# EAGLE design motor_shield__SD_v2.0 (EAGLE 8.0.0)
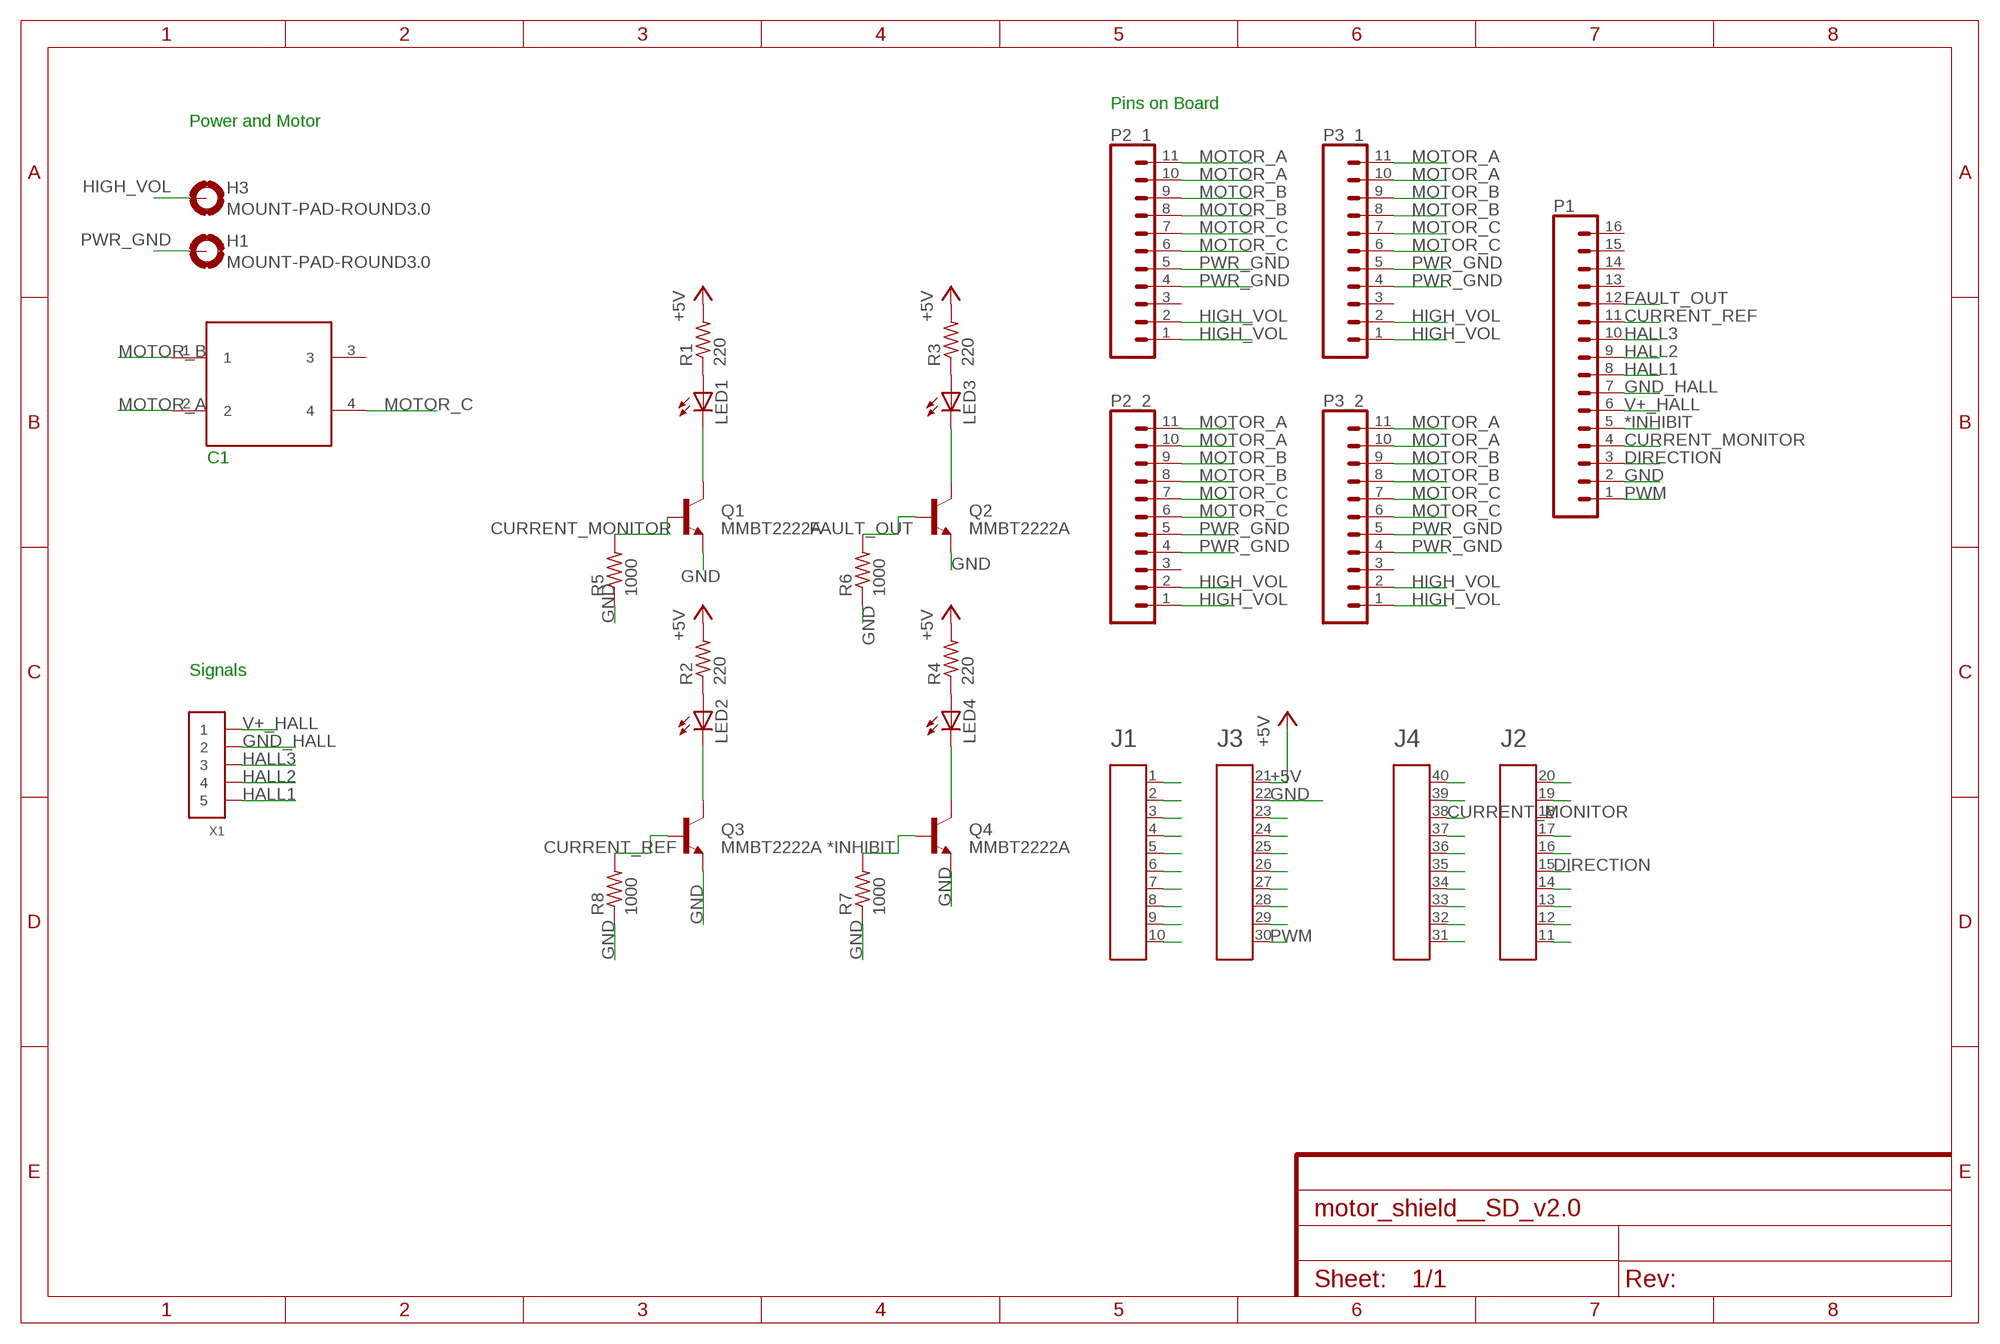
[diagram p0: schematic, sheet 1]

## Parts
A1  HEADER4X10-BOOSTERPACK  [4X10-BOOSTERPACK]
C1  MOLEX4CON  [MOLEX4CON]
H1  MOUNT-PAD-ROUND3.0  [3,0-PAD]
H3  MOUNT-PAD-ROUND3.0  [3,0-PAD]
LED1  LEDCHIPLED_0805  [CHIPLED_0805]
LED2  LEDCHIPLED_0805  [CHIPLED_0805]
LED3  LEDCHIPLED_0805  [CHIPLED_0805]
LED4  LEDCHIPLED_0805  [CHIPLED_0805]
P1  CONN_16LOCK  [1X16_LOCK]
P2_1  CONN_11  [1X11]
P2_2  CONN_11  [1X11]
P3_1  CONN_11  [1X11]
P3_2  CONN_11  [1X11]
Q1  MMBT2222A  TRANSISTOR_NPNMMBT2222A  [SOT23-3]
Q2  MMBT2222A  TRANSISTOR_NPNMMBT2222A  [SOT23-3]
Q3  MMBT2222A  TRANSISTOR_NPNMMBT2222A  [SOT23-3]
Q4  MMBT2222A  TRANSISTOR_NPNMMBT2222A  [SOT23-3]
R1  220  R-US_R0603  [R0603]
R2  220  R-US_R0603  [R0603]
R3  220  R-US_R0603  [R0603]
R4  220  R-US_R0603  [R0603]
R5  1000  R-US_R0603  [R0603]
R6  1000  R-US_R0603  [R0603]
R7  1000  R-US_R0603  [R0603]
R8  1000  R-US_R0603  [R0603]
X1  CONN_5-1-53261  [PB-53261-05]

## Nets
*INHIBIT: P1.5 Q4.1(B) R7.2
+5V: A1.21 R1.2 R2.2 R3.2 R4.2
CURRENT_MONITOR: A1.38 P1.4 Q1.1(B) R5.2
CURRENT_REF: P1.11 Q3.1(B) R8.2
DIRECTION: A1.15 P1.3
FAULT_OUT: P1.12 Q2.1(B) R6.2
GND: A1.22 P1.2 Q1.2(E) Q2.2(E) Q3.2(E) Q4.2(E) R5.1 R6.1 R7.1 R8.1
GND_HALL: P1.7 X1.2
HALL1: P1.8 X1.5
HALL2: P1.9 X1.4
HALL3: P1.10 X1.3
HIGH_VOL: H3.B3,0(MOUNT) P2_1.1 P2_1.2 P2_2.1 P2_2.2 P3_1.1 P3_1.2 P3_2.1 P3_2.2
MOTOR_A: C1.2 P2_1.10 P2_1.11 P2_2.10 P2_2.11 P3_1.10 P3_1.11 P3_2.10 P3_2.11
MOTOR_B: C1.1 P2_1.8 P2_1.9 P2_2.8 P2_2.9 P3_1.8 P3_1.9 P3_2.8 P3_2.9
MOTOR_C: C1.4 P2_1.6 P2_1.7 P2_2.6 P2_2.7 P3_1.6 P3_1.7 P3_2.6 P3_2.7
N$1: LED1.A R1.1
N$2: LED2.A R2.1
N$10: LED3.A R3.1
N$11: LED4.A R4.1
N$15: LED1.C Q1.3(C)
N$16: LED2.C Q3.3(C)
N$30: LED3.C Q2.3(C)
N$41: LED4.C Q4.3(C)
N$46: A1.1
N$47: A1.2
N$48: A1.3
N$49: A1.4
N$50: A1.5
N$51: A1.6
N$52: A1.7
N$53: A1.8
N$54: A1.9
N$55: A1.10
N$58: A1.23
N$59: A1.24
N$60: A1.25
N$61: A1.26
N$62: A1.27
N$63: A1.28
N$64: A1.29
N$66: A1.40
N$67: A1.39
N$69: A1.37
N$70: A1.36
N$71: A1.35
N$72: A1.34
N$73: A1.33
N$74: A1.32
N$75: A1.31
N$76: A1.20
N$77: A1.19
N$79: A1.17
N$80: A1.16
N$82: A1.14
N$83: A1.13
N$84: A1.12
N$85: A1.11
PWM: A1.30 P1.1
PWR_GND: H1.B3,0(MOUNT) P2_1.4 P2_1.5 P2_2.4 P2_2.5 P3_1.4 P3_1.5 P3_2.4 P3_2.5
V+_HALL: P1.6 X1.1
Unconnected: A1.18 C1.3 P1.13 P1.14 P1.15 P1.16 P2_1.3 P2_2.3 P3_1.3 P3_2.3

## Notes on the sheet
- Pins on Board
- Power and Motor
- C1
- Signals

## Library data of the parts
A1 = EAGLE_BoosterPack_Library:HEADER4X10-BOOSTERPACK
C1 = TREC1:MOLEX4CON
H1 H3 = holes:MOUNT-PAD-ROUND: MOUNTING PAD, round
LED1-LED4 = adafruit:LED: LED
P1 = SparkFun-Connectors:CONN_16: Multi connection point. Often used as Generic Header-pin footprint for 0.1 inch spaced/style header connections On any of the 0.1 inch spaced packages, you can populate with these: Break Away Headers - Straight (PRT-00116) Break Away Male Headers - Right Angle (PRT-00553) Female Headers (PRT-00115)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
P2_1 P2_2 P3_1 P3_2 = SparkFun-Connectors:CONN_11: Multi connection point. Often used as Generic Header-pin footprint for 0.1 inch spaced/style header connections On any of the 0.1 inch spaced packages, you can populate with these: Break Away Headers - Straight (PRT-00116) Break Away Male Headers - Right Angle (PRT-00553) Female Headers (PRT-00115)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
Q1-Q4 = SparkFun-DiscreteSemi:TRANSISTOR_NPN: Generic NPN BJT MMBT2222A - TRANS-08049 (SOT-23, 1A 40V) MPSA42 - TRANS-09116 (SOT-23, 500mA 300V) MMBT5088LT1G - TRANS-11160 (SOT-23, 50 mA 30V) BC547 - COM-08928 (TO-92 45V 100mA) (1.Collector 2.Base 3.Emitter) 2N3904 - COM-00521 (TO-92 40V 200mA) (1.Emitter 2.Base 3.Collector) P2N2222A -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; PROD_ID: TRANS-08049
R1-R8 = adafruit:R-US_: RESISTOR, American symbol
X1 = pel_molex:CONN_5-1

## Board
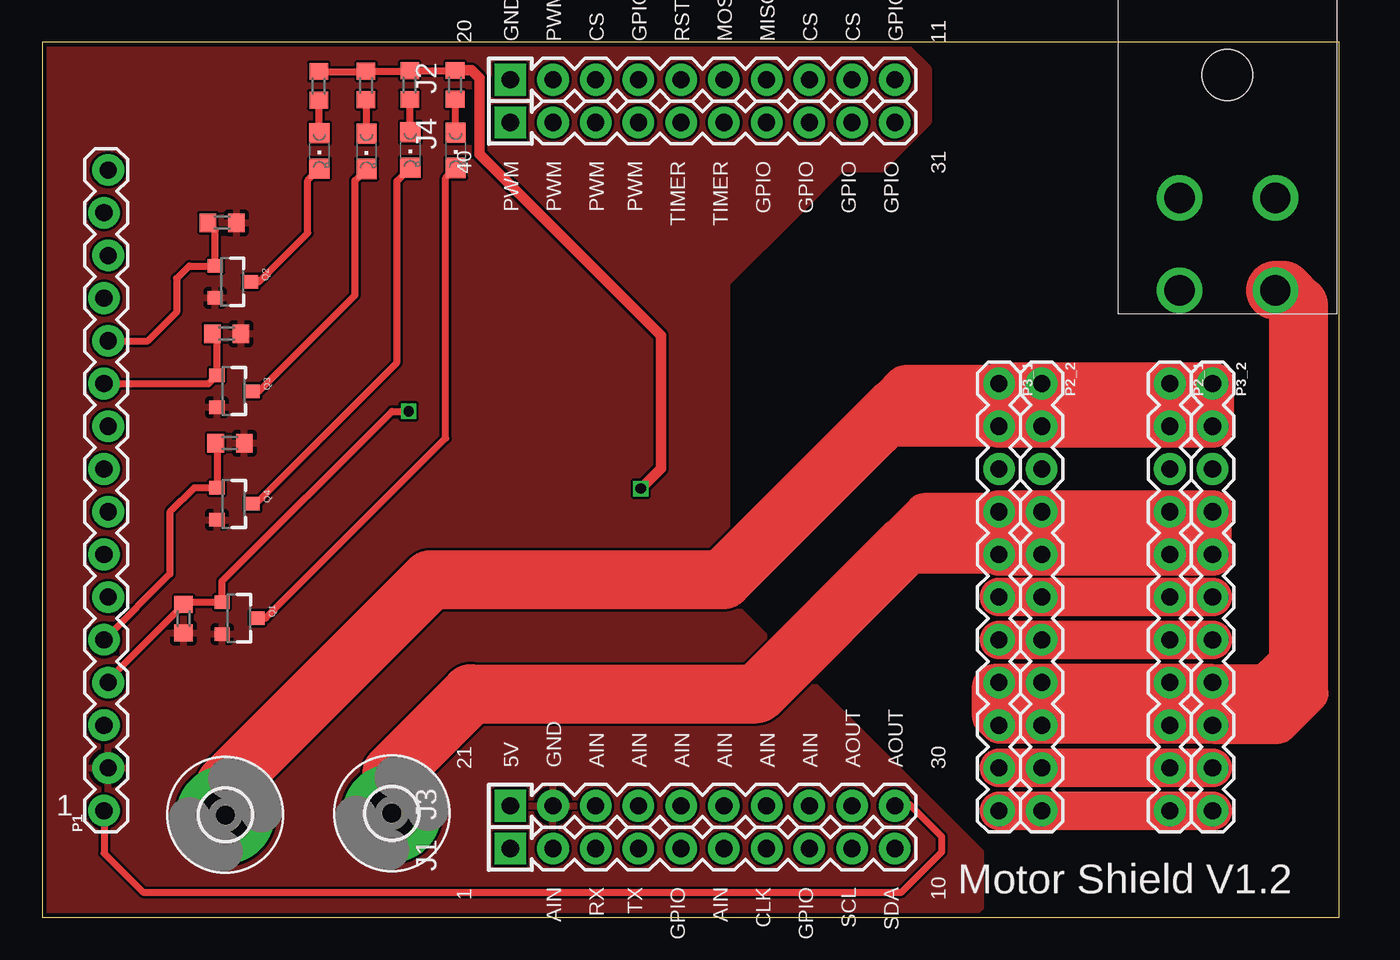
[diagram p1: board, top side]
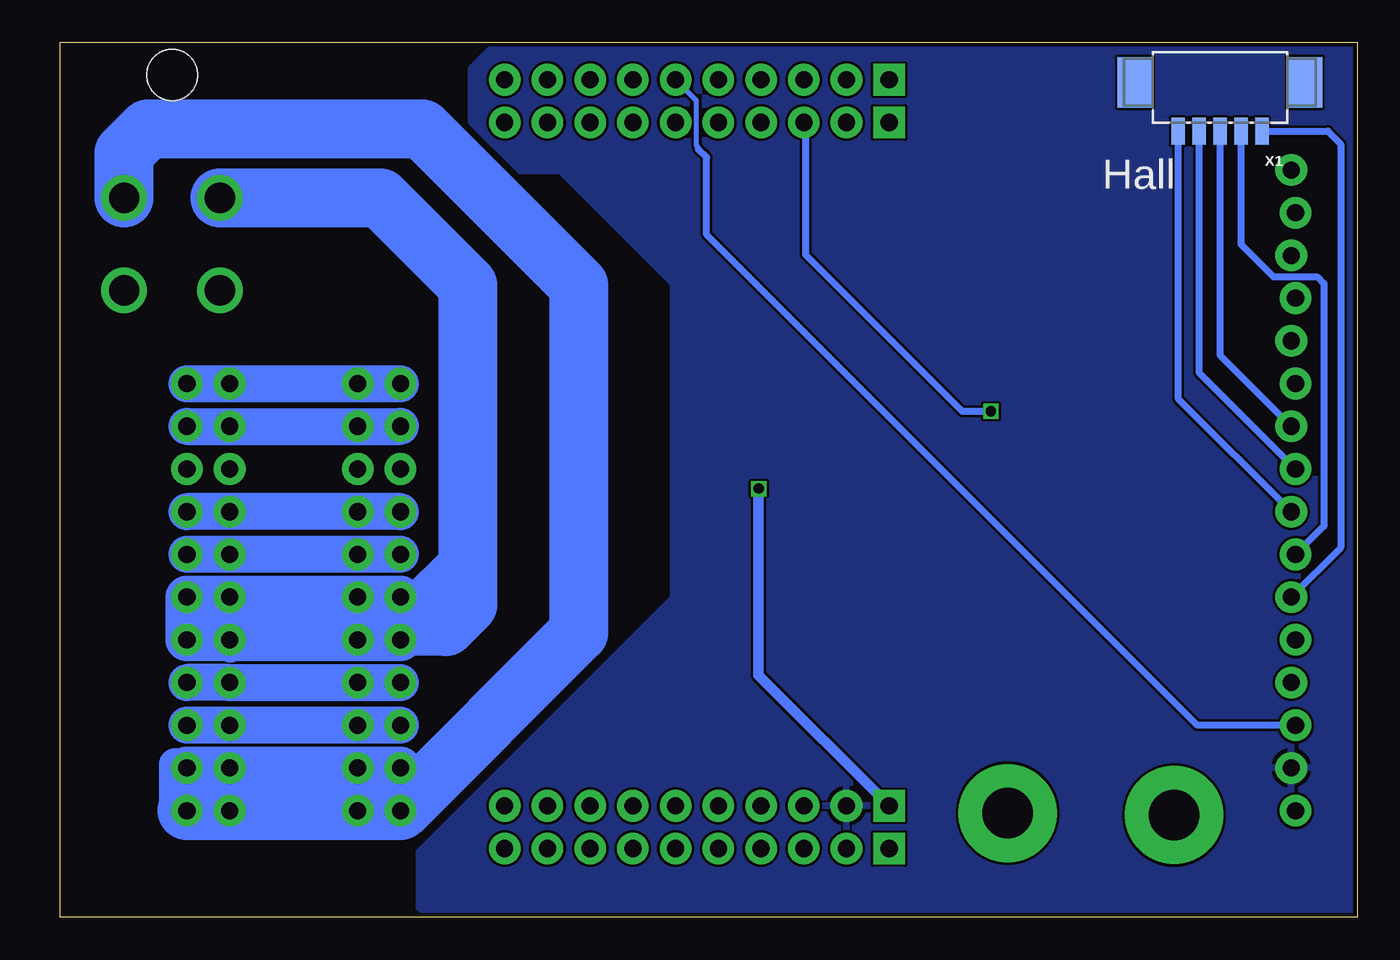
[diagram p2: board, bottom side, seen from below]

Size 77.14 x 52.06 mm. Coordinates in mm from the lower left corner, seen from the top.
Outline: 0,0 77.14,0 77.14,52.06 0,52.06 0,0
Copper layers (1*16): Top 0.035mm / dielectric 1.5mm / Bottom 0.035mm
Design rules "SeeedStudio_2layer_DRU_no_angle_20140221": minimum track width 6mil, minimum drill 12mil, track to track 6mil, track to pad 6mil, pad to pad 6mil, via to via 6mil, smd to smd 0mil, copper to edge 10mil, drill to drill 10mil, minimum pad ring 10mil, minimum via ring 6mil, stop-mask expansion 2mil, vias tented up to drill 100mil, thermal gap 10mil

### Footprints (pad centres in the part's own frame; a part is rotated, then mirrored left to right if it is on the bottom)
4X10-BOOSTERPACK = drill 1.016 pad 1.88 square: 1 0,10.16; 20 45.72,10.16; 21 2.54,10.16; 40 43.18,10.16 | drill 1.016 pad 1.88: 2 0,7.62; 3 0,5.08; 4 0,2.54; 5 0,0; 6 0,-2.54; 7 0,-5.08; 8 0,-7.62; 9 0,-10.16; 10 0,-12.7; 11 45.72,-12.7; 12 45.72,-10.16; 13 45.72,-7.62; 14 45.72,-5.08; 15 45.72,-2.54; 16 45.72,0; 17 45.72,2.54; 18 45.72,5.08; 19 45.72,7.62; 22 2.54,7.62; 23 2.54,5.08; 24 2.54,2.54; 25 2.54,0; 26 2.54,-2.54; 27 2.54,-5.08; 28 2.54,-7.62; 29 2.54,-10.16; 30 2.54,-12.7; 31 43.18,-12.7; 32 43.18,-10.16; 33 43.18,-7.62; 34 43.18,-5.08; 35 43.18,-2.54; 36 43.18,0; 37 43.18,2.54; 38 43.18,5.08; 39 43.18,7.62
MOLEX4CON = drill 1.8: 1 3.67,21.4; 2 3.67,15.9; 3 9.37,21.4; 4 9.37,15.9 | hole 3: 6.52,8.6
3,0-PAD = drill 3 pad 5.842: B3,0 0,0
CHIPLED_0805 = smd 1.2 x 1.2: A 0,-1.05; C 0,1.05
1X16_LOCK = drill 1.016 pad 1.88: 1 0,0.127; 2 2.54,-0.127; 3 5.08,0.127; 4 7.62,-0.127; 5 10.16,0.127; 6 12.7,-0.127; 7 15.24,0.127; 8 17.78,-0.127; 9 20.32,0.127; 10 22.86,-0.127; 11 25.4,0.127; 12 27.94,-0.127; 13 30.48,0.127; 14 33.02,-0.127; 15 35.56,0.127; 16 38.1,-0.127
1X11 = drill 1.016 pad 1.88: 1 0,0; 2 2.54,0; 3 5.08,0; 4 7.62,0; 5 10.16,0; 6 12.7,0; 7 15.24,0; 8 17.78,0; 9 20.32,0; 10 22.86,0; 11 25.4,0
SOT23-3 = smd 0.8 x 0.9: 1 -0.95,-1; 2 0.95,-1; 3 0,1.1
R0603 = smd 1 x 1.1: 1 -0.85,0; 2 0.85,0
PB-53261-05 = smd 0.8 x 1.6: 1 -2.5,1.1; 2 -1.25,1.1; 3 0,1.1; 4 1.25,1.1; 5 2.5,1.1 | smd 2.1 x 3: MNT1 -5.05,-1.8; MNT2 5.05,-1.8

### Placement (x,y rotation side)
A1  38,4.1 90 top
C1  77,58.7 180 top
H1  20.8,6.2 0 top
H3  10.9,6.1 0 top
LED1  24.59,45.63 180 top
LED2  19.29,45.57 180 top
LED3  16.49,45.59 180 top
LED4  21.89,45.65 180 top
P1  3.81,6.35 90 top
P2_1  67.06,31.75 270 top
P2_2  59.44,31.75 270 top
P3_1  56.9,31.75 270 top
P3_2  69.6,31.75 270 top
Q1  11.7,17.8 270 top
Q2  11.3,37.8 270 top
Q3  11.4,31.3 270 top
Q4  11.4,24.6 270 top
R1  24.56,49.52 90 top
R2  19.26,49.48 90 top
R3  16.46,49.46 90 top
R4  21.86,49.5 90 top
R5  8.41,17.77 90 top
R6  10.71,41.31 180 top
R7  11.18,28.21 180 top
R8  10.98,34.71 180 top
X1  8.18,47.86 180 bottom

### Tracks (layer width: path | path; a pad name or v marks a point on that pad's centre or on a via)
*INHIBIT
  Top 0.406: P1.5 7.6,20.43 7.6,24.1 9.05,25.55 Q4.1 10.4,28.14 R7.2
+5V  (via drill 0.6)
  Top 0.406: R3.2 19.26,50.31 R2.2 21.86,50.33 R4.2 24.56,50.35 R1.2
  Top 0.61: R1.2 25.53,50.37 26,49.9 26,45.4 36.8,34.6 36.8,26.7 v35.6,25.5
  Bottom 0.61: v35.6,25.5 35.6,14.4 A1.21
CURRENT_MONITOR  (via drill 0.6)
  Top 0.406: P1.4 3.94,14.14 R5.2 8.54,18.75 Q1.1 10.7,20 20.8,30.1 v21.8,30.1
  Bottom 0.406: v21.8,30.1 23.5,30.1 32.8,39.4 32.8,47.16 A1.38
CURRENT_REF
  Top 0.406: R8.2 10.4,34.44 Q3.1 9.9,31.75 P1.11
DIRECTION
  Bottom 0.305: 39.2,45.7 39.2,45.8 39.3,45.9 39.3,48.58 A1.15
  Bottom 0.406: P1.3 9.53,11.43 38.7,40.6 38.7,45.2 39.2,45.7
FAULT_OUT
  Top 0.406: P1.12 6.29,34.29 8,36 8,38 8.75,38.75 Q2.1 10.3,40.87 R6.2
GND
  pour Bottom: 0.1,51.9 51.3,51.9 52.7,50.5 52.7,47.3 49.8,44.4 47.4,44.4 40.7,37.7 40.7,19 55.8,3.9 55.8,0.6 55.2,0 0.1,0 0,0.1 0,51.8
  pour Top: 0.1,52 51.2,52 52.7,50.5 52.7,47.3 49.9,44.5 47.5,44.5 44.9,41.9 40.7,37.7 40.7,19 55.8,3.9 55.8,0.6 55.2,0 -0.1,0 -0.1,51.8
GND_HALL
  Bottom 0.406: X1.2 6.93,40.03 5,38.1 2.4,38.1 2,37.7 2,23.27 P1.7
HALL1
  Bottom 0.406: X1.5 10.68,30.87 P1.8
HALL2
  Bottom 0.406: X1.4 9.43,32.41 P1.9
HALL3
  Bottom 0.406: X1.3 8.18,33.45 P1.10
HIGH_VOL
  Top 2.184: P3_1.1 51.25,31.75 50.4,30.9 | 49.5,29.1 59.33,29.1 P2_2.2
  Top 2.54: P2_1.1 P3_1.1 P3_1.2 P2_2.2 | P2_2.2 P3_2.2 P3_2.1 P2_1.1 | P2_2.1 P2_2.2 | P2_1.2 P2_1.1
  Top 3.51: H3.B3,0 10.9,7.9 23.1,20.1 40.5,20.1 49.5,29.1 50.8,30.4 57.3,30.4 57.8,30.9 63.7,30.9 64.2,30.4 64.7,30.4 64.8,30.5 69,30.5
  Bottom 2.184: P3_2.1 P3_1.1 | P3_2.2 P3_1.2
MOTOR_A
  Top 2.3: P3_1.10 P3_2.10 | P3_1.11 P3_2.11
  Bottom 1.93: P3_2.11 69.6,8.4 70.3,9.1 70.3,6.1 70.2,6
  Bottom 2.3: 59.44,6.06 P2_2.10 P2_2.11 | P2_1.11 P3_2.10 P2_1.10
  Bottom 2.54: P3_1.11 P2_1.11 P3_2.11 | P3_1.10 P2_2.10 P3_2.10
  Bottom 3.51: P3_2.11 P3_1.11 46.3,16.95 46.3,37.6 55.6,46.9 71.9,46.9 73.33,45.47 C1.2
MOTOR_B
  Top 1.676: P2_2.8 58.44,13.97 56.4,11.93 | P3_1.8 P2_2.9 | P2_1.9 P3_2.9
  Top 2.184: 73.8,15 72.77,13.97 P3_2.8 P3_1.8 56.57,13.97 56.4,13.8 56.4,11.93 | 56.4,11.93 P3_1.9 P2_2.9 P3_2.9 73.53,11.43 75.4,13.3 | 56.4,11.93 69.13,11.93 69.9,12.7
  Top 3.51: C1.1 73.8,37.3 74.7,36.4 74.7,13.6 73.8,12.7 69.9,12.7 57.3,12.7
  Bottom 0.406: P3_2.8 P2_1.8
  Bottom 2.184: P3_1.8 P2_1.8 P3_2.8 | P3_1.9 P3_2.9
MOTOR_C
  Top 2.3: P3_1.6 P3_2.6 | P3_1.7 P3_2.7
  Bottom 1.676: P2_1.7 P3_2.7 | P3_2.6 69.6,18.6 67,16 67,16.1 68.1,17.2
  Bottom 1.93: 53.8,20 54.75,19.05 P3_1.6 55.85,19.05 53.9,21
  Bottom 2.54: 66.5,16.51 P3_2.7 P3_2.6 P2_1.6 | P2_2.7 66.5,16.51 | P3_1.7 P2_2.7 | P2_1.6 P3_1.6 P2_2.7 | P2_1.6 67.06,17.07 66.5,16.51 | P2_2.6 P2_2.7 | P2_1.6 P2_1.7
  Bottom 3.51: C1.4 58.1,42.8 52.9,37.6 52.9,18.6 54.2,17.3 60.9,17.3 61,17.2 68.1,17.2 68.7,17.8
N$1
  Top 0.406: R1.1 24.56,46.71 LED1.A
N$2
  Top 0.406: R2.1 19.26,46.65 LED2.A
N$10
  Top 0.406: R3.1 16.46,46.67 LED3.A
N$11
  Top 0.406: R4.1 21.86,46.73 LED4.A
N$15
  Top 0.406: LED1.C 24,43.98 24,28.5 13.3,17.8 Q1.3
N$16
  Top 0.406: LED2.C 18.6,43.82 18.6,37 12.9,31.3 Q3.3
N$30
  Top 0.406: LED3.C 15.8,43.84 15.8,40.7 12.9,37.8 Q2.3
N$41
  Top 0.406: LED4.C 21.1,43.8 21.1,33 12.7,24.6 Q4.3
PWM
  Top 0.406: P1.1 3.68,3.82 6,1.5 51.1,1.5 53.5,3.9 53.5,4.8 51.6,6.7 50.76,6.7 A1.30
PWR_GND
  Top 2.184: P3_1.4 52.43,24.13 50.8,22.5 | P3_2.4 P3_2.5
  Top 2.54: P2_2.5 P3_1.5 P3_1.4 P2_2.4 | P2_1.5 P2_2.5 | P3_2.5 P2_1.5 | P2_2.4 P3_2.4 68.08,22.62 P2_1.5 | P2_2.4 P2_2.5 | P2_1.4 P2_1.5
  Top 3.51: H1.B3,0 20.8,8.6 25.5,13.3 42.5,13.3 51.4,22.2 67.67,22.2 68.08,22.62
  Bottom 2.184: P3_1.4 P3_2.4 | P3_1.5 P3_2.5
V+_HALL
  Bottom 0.406: X1.1 1.76,46.76 1,46 1,21.99 P1.6

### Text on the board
tPlace: 1 | Motor Shield V1.2
bPlace: Hall

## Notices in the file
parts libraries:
SparkFun-Connectors: Licensing: Creative Commons ShareAlike 4.0 International - https://creativecommons.org/licenses/by-sa/4.0
